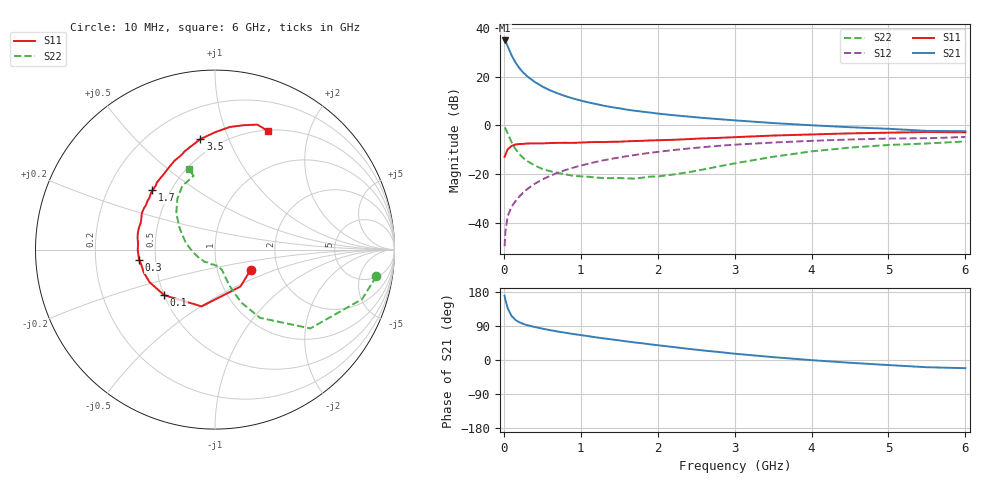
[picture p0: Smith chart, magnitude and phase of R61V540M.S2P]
! SIEMENS Small Signal Semiconductors
! BFR193
! Si NPN RF Bipolar Junction Transistor in SOT23
! VCE = 1.5 V  IC = 40 mA
! Common Emitter S-Parameters:  May  1996
# GHz  S  MA  R  50
!  f  S11  S21  S12  S22
! GHz  MAG  ANG  MAG  ANG  MAG  ANG  MAG  ANG
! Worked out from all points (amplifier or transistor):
!   36 points, 10 MHz to 6 GHz, reference 50 ohm
!   highest |S21| = 34.8 dB at 10 MHz (marker M1)
!   |S21| within 3 dB of that: start of sweep to 58.63 MHz
!   unconditionally stable (mu >= 1): 378.4 MHz to 1.899 GHz; 1.906 GHz to 2.032 GHz
!   at 250 MHz: K = 0.95, MSG = 24.6 dB, |S12| = -27.5 dB
!   at 1.4 GHz: K = 1.03, MAG = 9.6 dB, |S12| = -13.6 dB
!   at 6 GHz: K = 0.96, MSG = 1.2 dB, |S12| = -4.7 dB
!   S11 on the Smith chart (normalised r, x): 10 MHz: 1.44, -0.35; 100 MHz: 0.50, -0.30; 300 MHz: 0.40, -0.06; 1.7 GHz: 0.40, +0.34; 3.5 GHz: 0.40, +0.80; 6 GHz: 0.51, +1.42
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0.01  0.2282 -29.9  54.68 169.4  0.0034 81.6  0.9109 -9.4
0.02  0.2501 -55.5  52.28 159.4  0.0066 80.5  0.865 -18.6
0.05  0.3251 -103.3  41.66 136.7  0.0139 68.8  0.6891 -39.6
0.1  0.3804 -138.2  27.23 116.4  0.0218 65.1  0.4554 -56.6
0.15  0.4075 -153.6  19.48 106.0  0.0282 68.0  0.3314 -63.4
0.2  0.4169 -162.3  15.05 99.7  0.035 70.0  0.2628 -66.1
0.25  0.4191 -168.3  12.16 95.4  0.0423 71.5  0.2169 -68.0
0.3  0.4268 -172.4  10.23 92.1  0.0494 72.3  0.189 -68.8
0.4  0.4304 -179.5  7.786 87.2  0.0639 73.1  0.1525 -69.8
0.5  0.4298 175.5  6.241 82.8  0.0786 72.8  0.1292 -70.4
0.6  0.4368 171.1  5.236 78.8  0.0931 72.3  0.1163 -71.8
0.7  0.4401 167.4  4.523 75.1  0.1077 71.6  0.1074 -74.1
0.8  0.4411 163.9  3.975 71.9  0.1221 70.3  0.0999 -76.5
0.9  0.4398 160.3  3.557 68.6  0.137 69.2  0.0936 -78.5
1.1  0.4548 153.7  2.96 62.8  0.1655 66.7  0.0893 -86.9
1.4  0.4643 144.0  2.368 54.4  0.2078 62.3  0.0839 -100.3
1.7  0.4802 136.5  1.997 46.3  0.2484 57.8  0.0819 -119.0
2.2  0.5084 124.1  1.622 34.3  0.3134 49.9  0.0992 -150.8
3.5  0.6211 97.5  1.119 7.6  0.4473 28.7  0.2288 149.2
4.5  0.6886 83.0  0.92 -7.3  0.5163 14.5  0.3527 126.5
5.5  0.7354 71.2  0.774 -19.1  0.5474 0.8  0.4277 106.2
6  0.7231 65.9  0.764 -21.6  0.581 -3.2  0.4704 107.9
